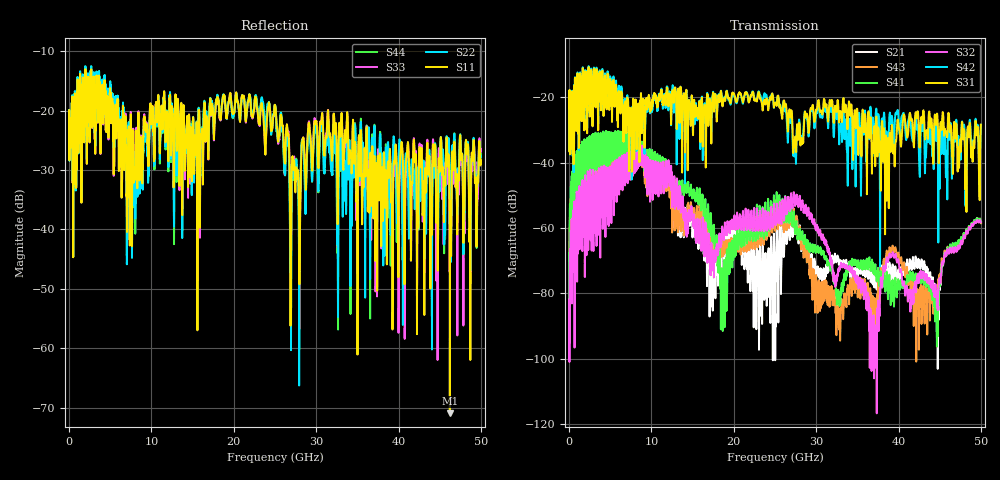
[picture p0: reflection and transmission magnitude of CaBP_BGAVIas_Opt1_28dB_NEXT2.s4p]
!* Samtec Inc. NovaRay Examax Flyover System  *
!*  REV DATE  = 08/08/18  *
!*  TYPE  = TOUCHSTONE  *
!*  PORTS  = 4 port  *
!*  UNITS  = GHz  *
!*  DATA RANGE = DC  to 50 GHz; 10 MHz Step  *
!*  PARAMETER  = S  *
!*  FORMAT  = Real-Imaginary  *
!*  REFERENCE  = 50 ohms  *
!*  SOURCE  = HFSS  *
!*  VALIDATED  = No  *
!*  MANUFACTURER = SAMTEC  *
!*  INTERCONNECT = NVAx to EBCx to EBCx to NVAx  *
!*  [Full Channel NVAx to EBCx to EBCx to NVAx  with PCB Trace and BGA Via]  *
!*  BOUNDARY A  = Silicon BGA Ball Pad  *
!*  BOUNDARY B  = Silicon BGA Ball Pad  *
!*  NVAx (end a) ->>- (end b) NVAx  *
!*  Port 01 ->>- Port 02  *
!*  Port 03 ->>- Port 04  *
!***************************** CHANNEL MODEL ******************************************
# GHz S RI R 50
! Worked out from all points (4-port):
!   5000 points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, 10 MHz to 50 GHz, reference 50 ohm
!   strongest paths, dB at 10 MHz, 12.51 GHz, 25.01 GHz, 37.51 GHz, 50 GHz:
!     S31: -23.1, -18.4, -21.9, -30.4, -28.3
!     S42: -23.1, -17.6, -21.8, -25.9, -28.4
!     S32: -85.5, -46.9, -58.4, -84.5, -58.3
!     S41: -72.0, -49.5, -57.7, -72.2, -58.2
!     S43: -75.7, -56.2, -60.7, -77.4, -58.5
!     S21: -76.8, -56.1, -80.3, -73.7, -58.0
!   lowest |S11| = -71.0 dB at 46.23 GHz (marker M1), VSWR 1.00, Z = 50 + j0.0275 ohm
!   |S11| at or under -10 dB: start of sweep to end of sweep
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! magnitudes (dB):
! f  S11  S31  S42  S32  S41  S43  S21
! 10 MHz  -21.9  -23.1  -23.1  -85.5  -72.0  -75.7  -76.8
! 1.66 GHz  -14.4  -11.3  -11.0  -50.6  -36.5  -41.0  -42.5
! 8.73 GHz  -24.6  -18.7  -20.3  -35.7  -34.3  -36.4  -35.8
! 18.57 GHz  -18.8  -21.4  -21.0  -61.6  -72.5  -65.5  -66.5
! 25.38 GHz  -25.2  -19.4  -19.5  -58.2  -57.3  -59.6  -77.1
! 46.23 GHz  -71.0  -30.6  -31.6  -66.7  -65.5  -66.3  -65.7
! 50 GHz  -28.4  -28.3  -28.4  -58.3  -58.2  -58.5  -58.0
